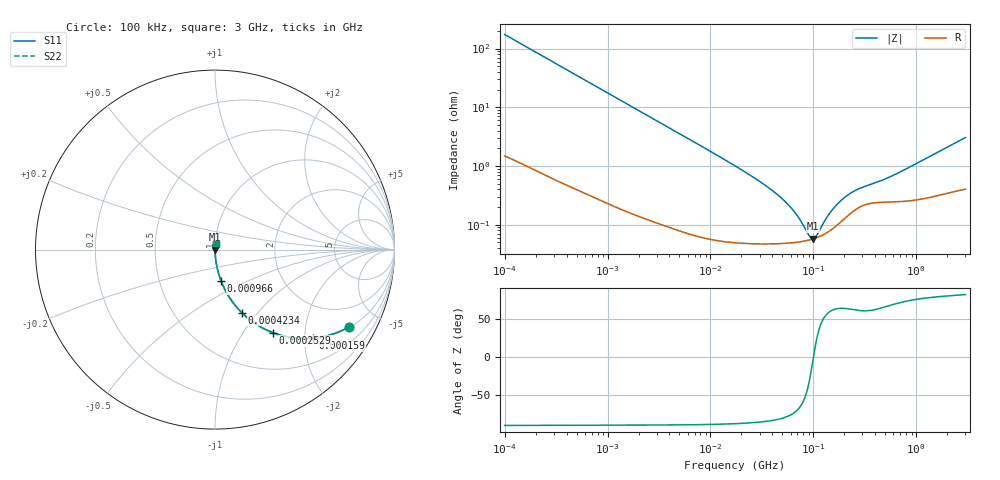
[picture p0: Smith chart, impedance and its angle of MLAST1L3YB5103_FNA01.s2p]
! MLAST1L3YB5103_FNA01  S-PARAMETER MODEL  ( Standard Model )
! Model Generated by TAIYO YUDEN Corporation (http://www.ty-top.com)
! Version 1.0
! TAIYO YUDEN Control No. 220601
! Copyright(c) 2010 TAIYO YUDEN CO.,LTD. All Rights Reserved.
! Product Description (link to TY-COMPAS)
! https://ds.yuden.co.jp/TYCOMPAS/or/detail?pn=MLAST1L3YB5103KFNA01&u=M
! Products Name : Multilayer Ceramic Capacitors
! Characteristics :
!  Capacitance : 0.01 [uF] , Rated Voltage : 25 [V] , TCC : B / X5R
!  Case Size : 1.0 x 0.5 / 0.039 x 0.02 [mm/inch] , Thickness : 0.3 / 0.012 [mm/inch]
!  (Conditions: Temperature = 25 [degC] , DC Bias Voltage = 0 [V])
! External Node Assignments :
!  1  o---| |---o  2
! GND o---------o GND
! Frequency Range : 100kHz  -  3GHz  [ 401 STEP ]
# MHZ S RI R 50
! Freq[MHz].  S11 Real  S11 Imag  S21 Real  S21 Imag  S12 Real  S12 Imag  S22 Real  S22 Imag
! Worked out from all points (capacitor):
!   401 points, 100 kHz to 3 GHz, reference 50 ohm
!   read as one part in series: C = 9.15 nF near 105.3 kHz
!   lowest |Z| = 57.5 mohm at 99.92 MHz (marker M1)
!   series resonance near 100.1 MHz, so ESL is about 280 pH
!   S11 on the Smith chart (normalised r, x): 100 kHz: 1.03, -3.47; 159 kHz: 1.02, -2.19; 252.9 kHz: 1.01, -1.38; 423.4 kHz: 1.01, -0.83; 966 kHz: 1.00, -0.36; 3 GHz: 1.01, +0.06
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0.1  0.7491 -0.4293  0.2509 0.4293  0.2509 0.4293  0.7491 -0.4293
0.159027  0.5449 -0.4934  0.4551 0.4934  0.4551 0.4934  0.5449 -0.4934
0.252895  0.3245 -0.4633  0.6755 0.4633  0.6755 0.4633  0.3245 -0.4633
0.423445  0.1489 -0.3505  0.8511 0.3505  0.8511 0.3505  0.1489 -0.3505
0.562235  0.0915 -0.2826  0.9085 0.2826  0.9085 0.2826  0.0915 -0.2826
0.965977  0.0343 -0.1757  0.9657 0.1757  0.9657 0.1757  0.0343 -0.1757
1.659646  0.0127 -0.105  0.9873 0.105  0.9873 0.105  0.0127 -0.105
3.161081  0.00417 -0.0559  0.9958 0.0559  0.9958 0.0559  0.00417 -0.0559
17.7727  0.000586 -0.00977  0.9994 0.00977  0.9994 0.00977  0.000586 -0.00977
33.85116  0.000493 -0.0047  0.9995 0.0047  0.9995 0.0047  0.000493 -0.0047
51.12795  0.000486 -0.00261  0.9995 0.00261  0.9995 0.00261  0.000486 -0.00261
66.15861  0.0005 -0.00154  0.9995 0.00154  0.9995 0.00154  0.0005 -0.00154
75.25761  0.000514 -0.00105  0.9995 0.00105  0.9995 0.00105  0.000514 -0.00105
90.13636  0.000547 -0.000382  0.9995 0.000382  0.9995 0.000382  0.000547 -0.000382
97.38194  0.000567 -0.0001  0.9994 0.0001  0.9994 0.0001  0.000567 -0.0001
99.92433  0.000575 -6.17e-06  0.9994 6.17e-06  0.9994 6.17e-06  0.000575 -6.17e-06
107.9567  0.000603 0.000276  0.9994 -0.000276  0.9994 -0.000276  0.000603 0.000276
147.0833  0.000807 0.00143  0.9992 -0.00143  0.9992 -0.00143  0.000807 0.00143
200.3904  0.00127 0.00261  0.9987 -0.00261  0.9987 -0.00261  0.00127 0.00261
273.0175  0.00194 0.00355  0.9981 -0.00355  0.9981 -0.00355  0.00194 0.00355
547.5153  0.00246 0.00596  0.9975 -0.00596  0.9975 -0.00596  0.00246 0.00596
3000  0.00491 0.03  0.9951 -0.03  0.9951 -0.03  0.00491 0.03
